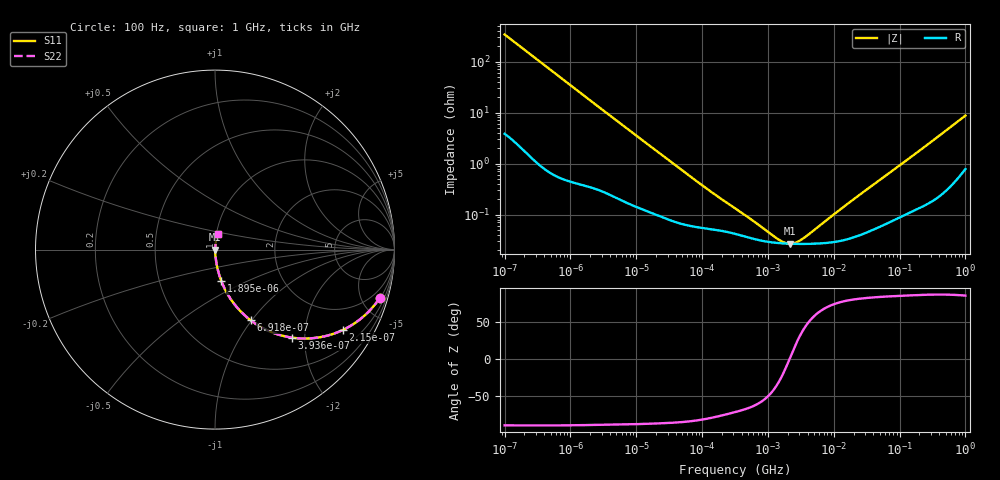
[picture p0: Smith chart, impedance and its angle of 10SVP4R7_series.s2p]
!  *** S-Parameter ***
!  Copyright (C) Panasonic Industry Corporation
!  Conductive Polymer Aluminum Soild Capacitor (OS-CON)
!  Parts No. 10SVP4R7M
!  Connection Mode : Series
!  1  o---||---o  2
!  GND o--------o GND
!  Conditions : Temperature = 20 degC  DC Bias = 0 V
! Frequency Range : 100Hz  -  1GHz  [ 401 Steps ]
# Hz S RI R 50
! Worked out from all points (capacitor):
!   401 points, 100 Hz to 1 GHz, reference 50 ohm
!   read as one part in series: C = 4.69 uF near 108.4 Hz
!   lowest |Z| = 26.9 mohm at 2.188 MHz (marker M1)
!   series resonance near 2.138 MHz, so ESL is about 1.2 nH
!   S11 on the Smith chart (normalised r, x): 100 Hz: 1.08, -6.77; 215 Hz: 1.03, -3.17; 393.6 Hz: 1.02, -1.74; 691.8 Hz: 1.01, -0.99; 1.895 kHz: 1.01, -0.36; 1 GHz: 1.02, +0.17
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100  0.9173 -0.2699  0.0827 0.2699  0.0827 0.2699  0.9173 -0.2699
149.6236  0.8351 -0.3656  0.1649 0.3656  0.1649 0.3656  0.8351 -0.3656
215.0305  0.7135 -0.4471  0.2865 0.4471  0.2865 0.4471  0.7135 -0.4471
296.8247  0.569 -0.4905  0.431 0.4905  0.431 0.4905  0.569 -0.4905
393.5501  0.4306 -0.4906  0.5694 0.4906  0.5694 0.4906  0.4306 -0.4906
691.831  0.1992 -0.3942  0.8008 0.3942  0.8008 0.3942  0.1992 -0.3942
994.2601  0.1093 -0.3057  0.8907 0.3057  0.8907 0.3057  0.1093 -0.3057
1487.647  0.0539 -0.2177  0.9461 0.2177  0.9461 0.2177  0.0539 -0.2177
1894.524  0.0351 -0.1747  0.9649 0.1747  0.9649 0.1747  0.0351 -0.1747
5188  0.00655 -0.0668  0.9934 0.0668  0.9934 0.0668  0.00655 -0.0668
22130.95  0.0012 -0.0162  0.9988 0.0162  0.9988 0.0162  0.0012 -0.0162
115478.2  0.000544 -0.00323  0.9995 0.00323  0.9995 0.00323  0.000544 -0.00323
316227.8  0.000422 -0.00126  0.9996 0.00126  0.9996 0.00126  0.000422 -0.00126
1404430  0.000278 -0.000185  0.9997 0.000185  0.9997 0.000185  0.000278 -0.000185
1788546  0.000271 -7.72e-05  0.9997 7.72e-05  0.9997 7.72e-05  0.000271 -7.72e-05
2187762  0.000268 9.99e-06  0.9997 -9.99e-06  0.9997 -9.99e-06  0.000268 9.99e-06
3019952  0.000266 0.000152  0.9997 -0.000152  0.9997 -0.000152  0.000266 0.000152
4704354  0.000268 0.000378  0.9997 -0.000378  0.9997 -0.000378  0.000268 0.000378
1.575796e7  0.000328 0.00154  0.9997 -0.00154  0.9997 -0.00154  0.000328 0.00154
6.99842e7  0.000745 0.00651  0.9993 -0.00651  0.9993 -0.00651  0.000745 0.00651
3.368992e8  0.0028 0.0294  0.9972 -0.0294  0.9972 -0.0294  0.0028 0.0294
1e9  0.015 0.0847  0.985 -0.0847  0.985 -0.0847  0.015 0.0847
